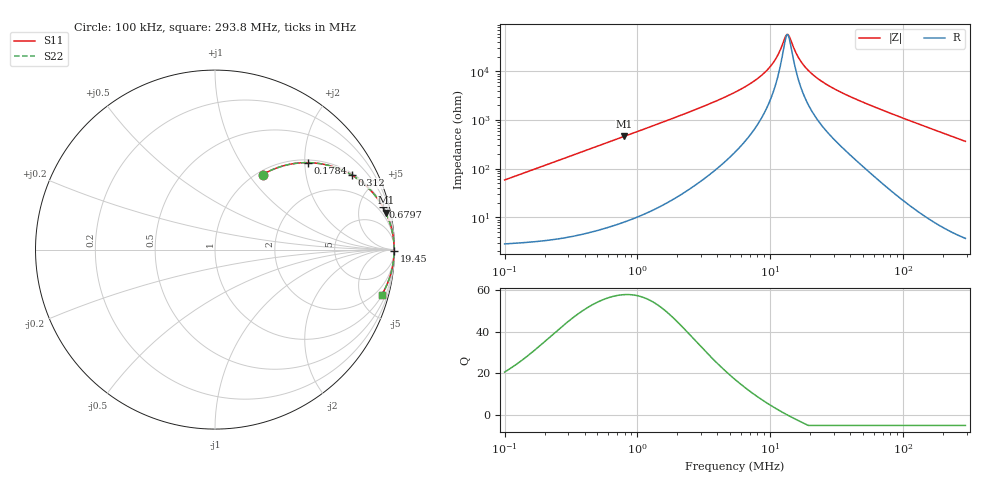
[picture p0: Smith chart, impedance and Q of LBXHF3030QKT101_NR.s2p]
! LBXHF3030QKT101_NR  S-PARAMETER MODEL  ( General Type )
! Model Generated by TAIYO YUDEN Corporation (http://www.ty-top.com)
! Version 1.0
! TAIYO YUDEN Control No. 210113NI43SB-FBB
! Copyright(c) 2021 TAIYO YUDEN CO.,LTD. All Rights Reserved.
! Product Description (link to TY-COMPAS)
! https://ds.yuden.co.jp/TYCOMPAS/or/detail?pn=LBXHF3030QKT101MNR&u=M
! Products Name : Inductors
! Characteristics :
!  Inductance : 100 uH , SRF(min) : 3.0 MHz , DC Resistance(max) : 2.028 Ohm
!  Rated Current : Saturation :210 mA , Temp Rise : 240 mA
!  Case Size : 3.0 x 3.0 / 0.118 x 0.118 [mm/inch] , Thickness : 1.5 / 0.059 [mm/inch]
!  (Conditions: Temperature = 25 degC , DC Bias Current/Voltage = 0A / 0V)
! External Node Assignments :
!  1  o---GGG---o  2
! GND o---------o GND
! Frequency Range : 0.1MHz  -  293.796821MHz  [ 402 STEP ]
# MHz S RI R 50
! Freq[MHz].  S11 Real  S11 Imag  S21 Real  S21 Imag  S12 Real  S12 Imag  S22 Real  S22 Imag
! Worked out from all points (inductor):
!   401 points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, 100 kHz to 293.8 MHz, reference 50 ohm
!   read as one part in series: L = 92.7 uH near 104.1 kHz
!   highest Q = 57.8 at 797.4 kHz (marker M1), where L = 92.2 uH
!   self-resonance near 13.31 MHz
!   S11 on the Smith chart (normalised r, x): 100 kHz: 1.06, +1.17; 178.4 kHz: 1.06, +2.08; 312 kHz: 1.08, +3.62; 679.7 kHz: 1.14, +7.88; 19.45 MHz: open; 293.8 MHz: 1.07, -7.29
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0.1  0.2648 0.4177  0.7352 -0.4177  0.7352 -0.4177  0.2648 0.4177
0.178416  0.5182 0.4845  0.4818 -0.4845  0.4818 -0.4845  0.5182 0.4845
0.31203  0.7616 0.4153  0.2384 -0.4153  0.2384 -0.4153  0.7616 0.4153
0.380976  0.8252 0.3699  0.1748 -0.3699  0.1748 -0.3699  0.8252 0.3699
0.679722  0.9358 0.2365  0.0642 -0.2365  0.0642 -0.2365  0.9358 0.2365
0.797429  0.952 0.2052  0.048 -0.2052  0.048 -0.2052  0.952 0.2052
1.451429  0.9841 0.116  0.0159 -0.116  0.0159 -0.116  0.9841 0.116
3.225526  0.9958 0.0504  0.0042 -0.0504  0.0042 -0.0504  0.9958 0.0504
5.420303  0.9977 0.0267  0.00228 -0.0267  0.00228 -0.0267  0.9977 0.0267
7.460113  0.9982 0.016  0.00184 -0.016  0.00184 -0.016  0.9982 0.016
9.479531  0.9983 0.00916  0.0017 -0.00916  0.0017 -0.00916  0.9983 0.00916
11.1211  0.9983 0.00491  0.00168 -0.00491  0.00168 -0.00491  0.9983 0.00491
12.78906  0.9983 0.00131  0.0017 -0.00131  0.0017 -0.00131  0.9983 0.00131
13.31002  0.9983 0.000289  0.00172 -0.000289  0.00172 -0.000289  0.9983 0.000289
14.13153  0.9983 -0.00124  0.00174 0.00124  0.00174 0.00124  0.9983 -0.00124
16.57869  0.9982 -0.00533  0.00183 0.00533  0.00183 0.00533  0.9982 -0.00533
19.44962  0.998 -0.00953  0.00197 0.00953  0.00197 0.00953  0.998 -0.00953
20.65007  0.998 -0.0112  0.00203 0.0112  0.00203 0.0112  0.998 -0.0112
25.21289  0.9977 -0.0169  0.00228 0.0169  0.00228 0.0169  0.9977 -0.0169
33.34297  0.9973 -0.0259  0.00275 0.0259  0.00275 0.0259  0.9973 -0.0259
78.67184  0.9931 -0.0706  0.00691 0.0706  0.00691 0.0706  0.9931 -0.0706
293.7968  0.9277 -0.2539  0.0723 0.2539  0.0723 0.2539  0.9277 -0.2539
